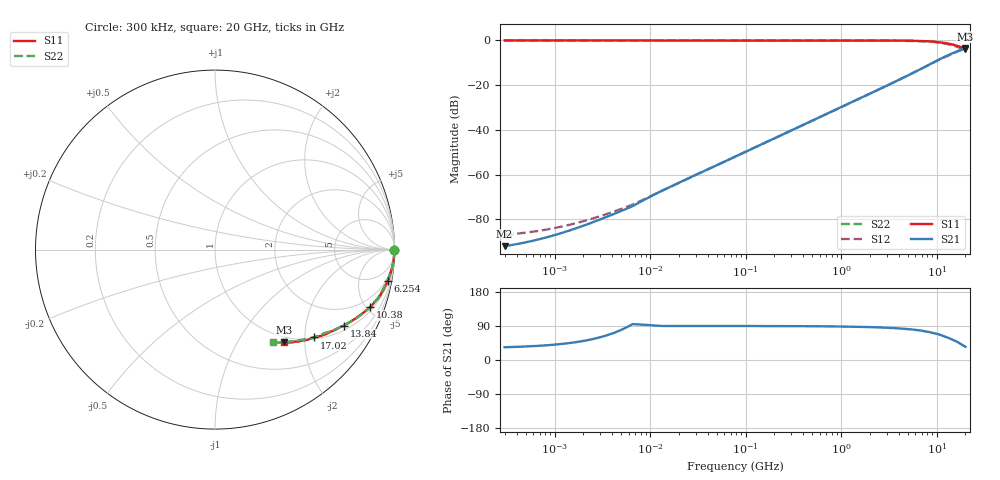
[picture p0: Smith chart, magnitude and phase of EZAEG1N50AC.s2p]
!*** S-Parameter ***
!Copyright (C)  Panasonic Industry
!ESD Suppressor
!Parts No.  EZAEG1N50AC
! Size : 0603mm
# hz S ma R 50
! 2 Port Network Data from SP1.SP block
! freq  magS11  angS11  magS21  angS21  magS12  angS12  magS22  angS22
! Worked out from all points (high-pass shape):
!   966 points, 300 kHz to 20 GHz, reference 50 ohm
!   highest |S21| = -3.55 dB at 20 GHz (marker M1); lowest = -92.1 dB at 300 kHz (marker M2)
!   |S21| within 3 dB of the highest: 13.4 GHz to end of sweep
!   lowest |S11| = -3.8 dB at 20 GHz (marker M3), VSWR 4.60, Z = 45.4 - j79.8 ohm
!   |S11| at or under -10 dB: nowhere
!   |S22| runs from -4.3 to 0.0 dB; largest |S21 - S12| = 0.018
!   S11 on the Smith chart (normalised r, x): 300 kHz: open; 6.254 GHz: 1, -11; 10.38 GHz: 1.27, -5.31; 13.84 GHz: 1.18, -3.28; 17.02 GHz: 1.04, -2.23; 20 GHz: 0.91, -1.60
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300000  1 0.0  2.493e-05 33.7  4.472e-05 -4.7  0.9999 0.0
1913988  1 0.0  6.901e-05 49.4  8.782e-05 18.4  0.9999 0.0
2381868  0.9999 0.0  8.179e-05 54.0  0.0001003 25.0  0.9999 0.0
2930201  0.9999 0.0  9.677e-05 59.3  0.000115 32.9  0.9999 0.0
3176065  0.9999 0.0  0.0001035 61.7  0.0001215 36.4  0.9999 0.0
6409445  1 -0.0  0.0001918 93.3  0.0002079 82.5  1 -0.0
1.221117e7  1 -0.0  0.000397 90.3  0.0003962 89.5  1 -0.0
7.790674e7  0.9998 -0.1  0.002513 89.7  0.00252 89.7  1 -0.1
4.970419e8  0.9997 -0.7  0.01598 89.1  0.01599 89.0  0.9998 -0.8
1.449732e9  0.9988 -2.0  0.0466 87.6  0.0466 87.5  0.9986 -2.3
2.219453e9  0.9973 -3.2  0.07148 86.4  0.0715 86.2  0.9965 -3.6
3.171107e9  0.9946 -4.7  0.1027 84.9  0.1025 84.6  0.9924 -5.3
4.583263e9  0.9883 -7.1  0.1503 82.2  0.15 81.9  0.9842 -7.9
6.253803e9  0.9775 -10.3  0.2091 78.9  0.2081 78.6  0.9703 -11.4
8.435577e9  0.9556 -15.2  0.2921 73.5  0.2885 73.2  0.9451 -16.9
1.037754e10  0.921 -20.2  0.3665 68.1  0.3596 67.2  0.9036 -22.5
1.205257e10  0.8815 -25.0  0.428 62.1  0.4189 61.9  0.8565 -27.7
1.383777e10  0.8336 -30.5  0.4891 56.4  0.4814 56.6  0.8029 -33.8
1.534815e10  0.7902 -35.4  0.5363 51.3  0.5277 50.9  0.7564 -38.9
1.702338e10  0.738 -41.5  0.5921 45.4  0.5806 45.6  0.7018 -45.6
1.910005e10  0.6738 -50.1  0.6439 38.0  0.6299 38.1  0.6348 -54.4
2e10  0.6426 -53.4  0.6646 34.8  0.6491 34.8  0.609 -57.9
